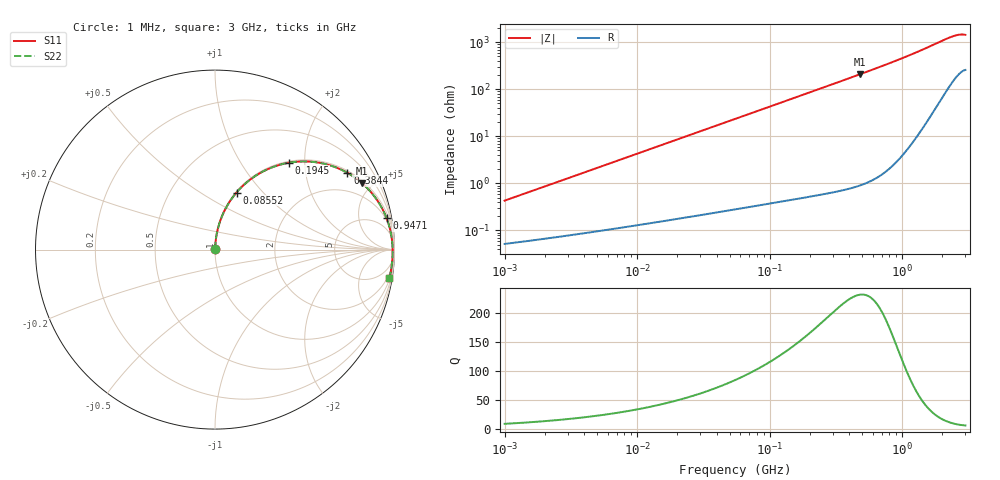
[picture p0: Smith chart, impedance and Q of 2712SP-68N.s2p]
# MHz  S  MA  R  50
!Freq  MagS11  AngS11  MagS21  AngS21  MagS12  AngS12  MagS22  AngS22
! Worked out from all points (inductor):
!   801 points, 1 MHz to 3 GHz, reference 50 ohm
!   read as one part in series: L = 67.9 nH near 1.041 MHz
!   highest Q = 231 at 479.2 MHz (marker M1), where L = 69 nH
!   S11 on the Smith chart (normalised r, x): 1 MHz: 1.00, +0.01; 85.52 MHz: 1.01, +0.73; 194.5 MHz: 1.03, +1.67; 384.4 MHz: 1.08, +3.40; 947.1 MHz: 2, +11; 3 GHz: 1, -12
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1  0.004268 82.8  0.9995 -0.2  0.9995 -0.2  0.004268 82.8
3.829105  0.01624 86.0  0.999 -0.9  0.999 -0.9  0.01624 86.0
8.037227  0.03403 86.1  0.9983 -2.0  0.9983 -2.0  0.03403 86.1
14.51587  0.06135 85.0  0.9966 -3.6  0.9966 -3.6  0.06135 85.0
29.56635  0.1241 81.8  0.9902 -7.2  0.9902 -7.2  0.1241 81.8
55.02866  0.2267 76.1  0.9713 -13.3  0.9713 -13.3  0.2266 76.1
85.51725  0.34 69.3  0.9372 -20.1  0.9372 -20.1  0.34 69.3
104.492  0.404 65.4  0.9113 -24.1  0.9113 -24.1  0.404 65.4
127.677  0.4749 60.8  0.8764 -28.7  0.8764 -28.7  0.4749 60.8
160.7668  0.5621 54.9  0.8232 -34.7  0.8232 -34.7  0.5621 54.9
194.4798  0.6353 49.6  0.7684 -40.0  0.7684 -40.0  0.6352 49.6
208.6098  0.6617 47.6  0.7459 -42.0  0.7459 -42.0  0.6616 47.6
278.9507  0.7634 39.1  0.642 -50.6  0.642 -50.6  0.7633 39.1
384.3922  0.8531 30.1  0.518 -59.7  0.518 -59.7  0.853 30.1
479.1891  0.8985 24.4  0.4351 -65.4  0.4351 -65.4  0.8984 24.4
609.4559  0.9344 18.8  0.3523 -70.9  0.3523 -70.9  0.9342 18.8
790.8254  0.9602 13.6  0.2741 -76.1  0.2741 -76.1  0.96 13.6
947.1245  0.9722 10.3  0.2274 -79.2  0.2274 -79.2  0.9719 10.3
1532.067  0.9881 2.6  0.1304 -85.8  0.1304 -85.8  0.9879 2.6
2357.171  0.9892 -4.3  0.07578 -88.4  0.07578 -88.4  0.9892 -4.3
2685.098  0.9873 -6.8  0.06819 -88.3  0.06819 -88.3  0.9875 -6.8
3000  0.9846 -9.3  0.06834 -88.9  0.06834 -88.9  0.985 -9.3
